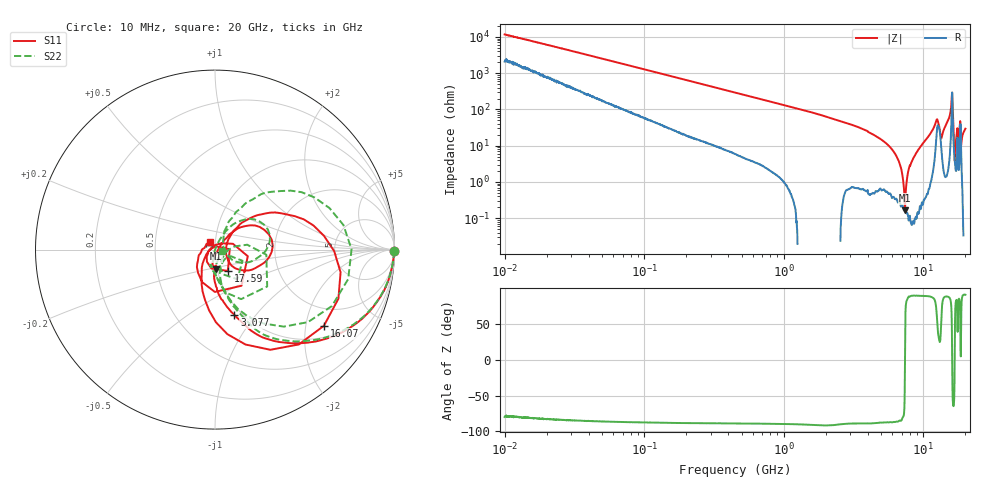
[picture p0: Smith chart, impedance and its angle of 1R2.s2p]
!Keysight Technologies,P5008B,MY61100088,A.16.20.02
!Date: Monday, October 30, 2023 16:11:21
!Correction: S11(C  2-Port  )
!S21(C  2-Port  )
!S12(C  2-Port  )
!S22(C  2-Port  )
!S2P File: Measurements: S11, S21, S12, S22:Log Frequency Sweep
# Hz S  dB  R 50
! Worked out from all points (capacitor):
!   1601 points, 10 MHz to 20 GHz, reference 50 ohm
!   read as one part in series: C = 1.36 pF near 10.39 MHz
!   lowest |Z| = 164 mohm at 7.375 GHz (marker M1)
!   series resonance near 7.381 GHz, so ESL is about 340 pH
!   S11 on the Smith chart (normalised r, x): 10 MHz: open; 3.077 GHz: 0.92, -0.79; 16.07 GHz: 1.35, -2.54; 17.59 GHz: 1.12, -0.27; 20 GHz: 0.95, +0.08
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1e7  -0.01 -0.5  -41.34 79.2  -41.33 79.1  -0.01 -0.5
3.555162e7  -0.02 -1.7  -30.89 83.5  -30.89 83.5  -0.02 -1.6
1.263918e8  -0.08 -5.8  -20.19 82.0  -20.20 82.0  -0.08 -5.7
4.472136e8  -0.54 -19.6  -9.85 69.5  -9.85 69.5  -0.54 -19.1
1.589917e9  -3.76 -53.1  -2.29 38.4  -2.30 38.4  -3.77 -51.6
3.077169e9  -8.41 -73.4  -0.76 18.1  -0.76 18.1  -8.44 -68.9
5.652411e9  -15.11 -90.6  -0.16 1.1  -0.16 1.1  -15.10 -83.0
7.375132e9  -19.42 -88.1  -0.05 -6.1  -0.05 -6.1  -19.47 -100.7
9.531902e9  -24.27 -100.3  -0.00 -14.4  -0.01 -14.5  -24.42 -99.2
1.004325e10  -27.68 -92.5  0.00 -16.5  -0.00 -16.5  -27.79 -101.5
1.068304e10  -36.00 -17.7  -0.01 -19.4  -0.01 -19.4  -53.65 -89.8
1.099193e10  -29.49 34.7  -0.03 -21.1  -0.03 -21.1  -32.01 65.8
1.147208e10  -21.73 45.4  -0.10 -24.1  -0.11 -24.2  -22.40 62.8
1.226101e10  -11.66 31.0  -1.04 -33.0  -1.05 -33.0  -11.78 41.8
1.27966e10  -11.02 -15.5  -2.67 -22.1  -2.67 -22.1  -11.34 -4.4
1.380717e10  -21.80 31.7  -0.21 -22.6  -0.22 -22.7  -21.74 54.3
1.525565e10  -8.62 33.8  -0.90 -42.5  -0.90 -42.5  -8.46 51.5
1.607405e10  -2.61 -35.0  -12.23 -19.7  -12.23 -19.8  -2.38 -12.5
1.66967e10  -12.26 -106.4  -0.76 -10.7  -0.76 -10.7  -11.82 -75.9
1.75924e10  -17.16 -58.8  -1.53 -23.0  -1.53 -23.0  -13.69 -53.0
1.889175e10  -17.97 -141.6  -0.26 -26.0  -0.27 -26.0  -17.06 -88.4
2e10  -25.98 120.4  -0.02 -34.7  -0.02 -34.8  -28.04 -10.5
